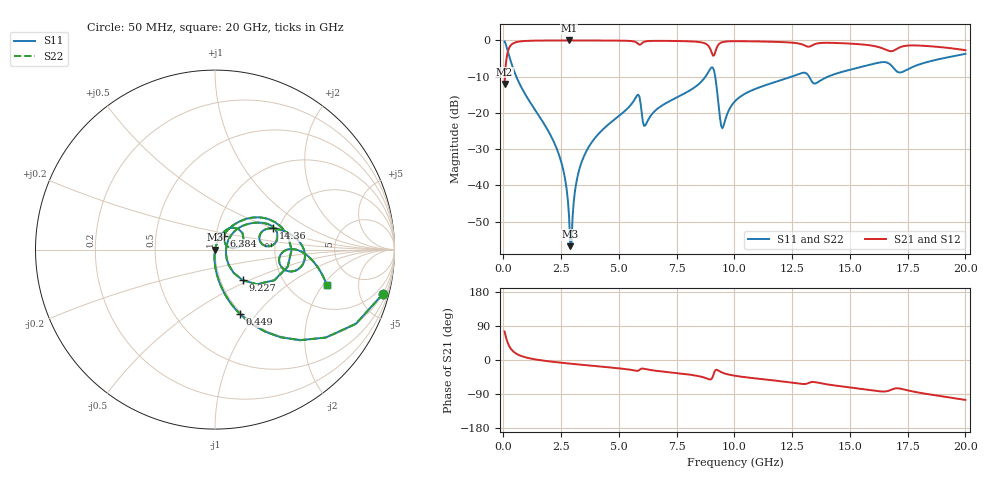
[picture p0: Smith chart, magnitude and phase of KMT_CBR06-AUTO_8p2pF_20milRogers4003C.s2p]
! Data measured by Modelithics Inc. support@modelithics.com 813-866-6335
! KEMET CBR06-AUTO 8.2pF, Pad Width= 0.851mm, Pad Length= 0.64mm, Pad Gap= 0.62mm, 20mil Rogers 4003C substrate Data, January 2022
# hz S ma R 50
! 2 Port Network Data from SP1.SP block
! freq  magS11  angS11  magS21  angS21  magS12  angS12  magS22  angS22
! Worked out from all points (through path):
!   401 points, 50 MHz to 20 GHz, reference 50 ohm
!   highest |S21| = -0.01 dB at 2.843 GHz (marker M1); lowest = -12.0 dB at 50 MHz (marker M2)
!   group delay of S21, straight-line fit = 15.4 ps
!   lowest |S11| = -56.8 dB at 2.893 GHz (marker M3), VSWR 1.00, Z = 50.1 - j0.129 ohm
!   |S11| at or under -10 dB: 557.7 MHz to 8.745 GHz (8.188 GHz wide, 176 % of centre); 9.167 GHz to 12.48 GHz (3.309 GHz wide, 30.6 % of centre); 13.23 GHz to 14.05 GHz (812.9 MHz wide, 5.96 % of centre)
!   |S22| runs from -56.8 to -0.3 dB; largest |S21 - S12| = 0
!   S11 on the Smith chart (normalised r, x): 50 MHz: 0.98, -7.62; 449 MHz: 0.98, -0.83; 6.384 GHz: 1.09, +0.17; 9.227 GHz: 1.27, -0.46; 14.36 GHz: 1.87, +0.50; 20 GHz: 3.17, -2.17
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5e7  0.9679 -14.7  0.2512 75.3  0.2512 75.3  0.9679 -14.7
2.495e8  0.6083 -53.3  0.7931 36.6  0.7931 36.6  0.6083 -53.3
4.49e8  0.3866 -68.7  0.9216 21.2  0.9216 21.2  0.3866 -68.7
2.34425e9  0.02992 -94.7  0.9987 -6.2  0.9987 -6.2  0.02992 -94.7
2.6435e9  0.01353 -94.6  0.999 -8.1  0.999 -8.1  0.01353 -94.6
2.843e9  0.003657 -85.7  0.999 -9.4  0.999 -9.4  0.003657 -85.7
2.892875e9  0.001451 -62.8  0.999 -9.7  0.999 -9.7  0.001451 -62.8
3.391625e9  0.02128 74.8  0.9987 -12.6  0.9987 -12.6  0.02128 74.8
5.785625e9  0.1742 40.6  0.925 -28.8  0.925 -28.8  0.1742 40.6
6.13475e9  0.06674 37.3  0.966 -23.9  0.966 -23.9  0.06674 37.3
6.384125e9  0.09229 56.3  0.9843 -26.6  0.9843 -26.6  0.09229 56.3
6.73325e9  0.1184 57.8  0.9869 -29.3  0.9869 -29.3  0.1184 57.8
8.977625e9  0.4143 10.3  0.7338 -51.3  0.7338 -51.3  0.4143 10.3
9.227e9  0.2299 -47.9  0.7829 -25.7  0.7829 -25.7  0.2299 -47.9
9.476375e9  0.06148 -1.7  0.9468 -33.4  0.9468 -33.4  0.06148 -1.7
1.0025e10  0.145 43.2  0.976 -41.6  0.976 -41.6  0.145 43.2
1.291775e10  0.355 18.4  0.8838 -63.2  0.8838 -63.2  0.355 18.4
1.336662e10  0.2665 6.1  0.8537 -57.9  0.8537 -57.9  0.2665 6.1
1.436412e10  0.3449 20.1  0.9229 -67.3  0.9229 -67.3  0.3449 20.1
1.670825e10  0.4758 -13.4  0.7134 -80.5  0.7134 -80.5  0.4758 -13.4
1.785538e10  0.4487 0.1  0.8526 -84.6  0.8526 -84.6  0.4487 0.1
2e10  0.6525 -17.5  0.7325 -105.3  0.7325 -105.3  0.6525 -17.5
